VAR_GLOBAL
	
//	inputs 	AT%IB0 : ARRAY[0..200] OF BYTE;	// define used input space - not used
//	outputs AT%QB0 : ARRAY[0..200] OF BYTE;	// define used output space - not used
	memory 	AT%MB0 : ARRAY[0..200] OF BYTE;	// define used memory space
//	data	: ARRAY[0..200] OF BYTE;		// define used data space - not used


//Datapoints SLAVE -> MASTER (monitoring direction)
	(* Input IB0-99*)	// example

	(* Output QB0-99*)	// example
	
	(* Memory MB0-99*)	// example
		(*Single points*)
		bSlaveToMaster 		AT%MX0.0	: BOOL;			// obj addr: 10 - M_SP_NA_1 at byte/bit offset: 0/0
		
		(*Bitstrings*)
		nBitstring 			AT%MD1		: DWORD;		// obj addr: 11 - M_BO_TB_1	at byte offset: 4 (AT%MD1 -> 4*1)	
		
		(*Measurement Value*)
		// scaled value
		nMeasurementValue 	AT%MW10		: INT;			// obj addr: 12 - M_ME_NB_1 at byte offset: 20 (AT%MW10 -> 2*10)
		// short floating point value	
		fMeasurementValue 	AT%MD6		: REAL;			// obj addr: 13 - M_ME_NC_1 at byte offset: 24 (AT%MD6 -> 4*6)
		
		(*Integrated totals*)
		nCounter 			AT%MD10		: DWORD :=0;	// obj addr: 200 - M_IT_NA_1 at byte offset: 40 (AT%MD10 -> 4*10):
		
	(* Data *)
	
//Datapoints MASTER -> SLAVE (control directon)
	(* Input IB100-200*)	// example

	(* Output QB100-200*)	// example
	
	(* Memory MB100-200*)	// example
		(*Single points*)
		bMasterToSlave 		AT%MX100.0	: BOOL;			// obj addr: 101 - C_SC_NA_1 at byte/bit offset: 100/0
		
	(* Data *)
	
//other variables
		
END_VAR
